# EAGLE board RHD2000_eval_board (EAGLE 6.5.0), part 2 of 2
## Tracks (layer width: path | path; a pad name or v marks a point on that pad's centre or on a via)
+3V3  (via drill 0.25)
  Top 0.381: BRD1.JP2-2 33.93,34.95 34.54,34.95 BRD1.JP2-4 34.75,34.95 35.36,34.95 BRD1.JP2-6 35.56,34.75 35.56,30.07 34.75,29.26 24.18,29.26 24.18,30.48 +3.3V_FPGA_1.1 | BRD1.JP3-9 37.19,81.08 37.8,81.08 BRD1.JP3-11 38,81.08 38.61,81.08 BRD1.JP3-13 38.81,81.08 v38.81,79.65
  Bottom 0.381: v38.81,79.65 44.3,74.17 44.3,65.63 | 44.3,65.63 52.63,65.63 53.65,64.62 77.42,64.62 +3.3V_FPGA_2.1 | 44.3,65.63 31.09,65.63 31.09,37.39 24.18,30.48 +3.3V_FPGA_1.1
+3V3ADC  (via drill 0.25)
  Top 0.381: C20.1 134.31,84.94 v134.31,83.92 134.31,82.7 U10.1 134.11,82.5 134.11,81.89 133.71,81.48 128.83,81.48 128.73,81.58 | C19.1 129.24,84.94 129.24,82.7 U9.1 129.03,82.5 129.03,81.89 128.73,81.58 | C18.1 124.16,84.94 124.16,82.7 U8.1 123.95,82.5 123.95,81.89 123.65,81.58 | C16.1 114,84.94 114,82.7 U6.1 114,82.5 116.43,82.5 116.43,81.89 116.84,81.48 118.87,81.48 | C17.1 119.08,84.94 119.08,82.7 U7.1 118.87,82.5 118.87,81.48 | 123.65,81.58 123.55,81.48 118.87,81.48 | 128.73,81.58 128.63,81.48 123.75,81.48 123.65,81.58 | C15.1 108.92,84.94 v108.92,83.92 108.92,82.7 U5.1 108.71,82.5 108.71,81.89 108.31,81.48 103.63,81.48 | C13.1 98.75,84.94 98.75,82.7 U3.1 98.75,82.5 101.19,82.5 101.19,81.89 101.6,81.48 103.63,81.48 | C14.1 103.83,84.94 103.83,82.7 U4.1 103.63,82.5 103.63,81.48 | 87.58,81.08 84.94,81.08 U2.5 | 87.58,81.08 87.58,79.65 C12.1 | 87.58,81.08 90.83,81.08 90.83,88.8 94.69,92.66 S2.2
  pour Route3: 73.66,97.79 138.43,97.79 138.43,77.47 73.66,77.47
+3V3DAC  (via drill 0.25)
  Top 0.381: 89,30.89 89,31.29 U14.2 | 89,30.89 C32.1 | 89,30.89 U14.1 88.8,30.68 87.99,29.87 87.99,26.21 88.09,26.11 | 89,23.37 89,23.77 U12.2 88.8,23.77 87.99,23.77 87.99,26.01 88.09,26.11 | 89,23.37 89,23.16 U12.1 | 89,23.37 92.66,23.37 C30.1 92.86,23.16 95.5,23.16 95.5,22.55 95.91,22.15 97.54,22.15 97.54,20.52 97.33,20.32 95.5,20.32 95.5,19.3 | 89,27.23 89,27.43 U13.2 | 89,27.23 89,27.03 U13.1 88.8,26.82 88.09,26.11 | 89,27.23 92.66,27.23 C31.1 | U11.1 89,19.51 89,19.91 U11.2 | U11.1 89.2,19.51 92.66,19.51 C29.1 92.86,19.3 95.5,19.3 | 104.55,22.86 104.44,22.96 104.44,29.26 105.26,30.07 C45.1 105.46,30.07 105.46,33.12 112.37,33.12 112.57,32.92 112.57,32.51 112.98,32.11 U22.4 | 104.55,22.86 R13.1 | 95.5,19.3 95.5,18.9 95.91,18.49 104.44,18.49 104.44,22.76 104.55,22.86 | U19.5 111.56,41.66 v113.59,41.66 115.42,41.66 C23.1 115.62,41.45 119.89,37.19 119.89,30.68 120.5,30.07 C46.1 | 89,46.13 89,46.53 U18.2 | 89,46.13 v90.83,46.13 C36.1 | 89,46.13 U18.1 | 89,42.47 89,42.67 U17.2 | 89,42.47 89,42.27 U17.1 | 89,42.47 v90.83,42.47 92.66,42.47 C35.1 | 89,38.61 89,39.01 U16.2 | 89,38.61 89,38.41 U16.1 | 89,38.61 v90.83,38.61 92.66,38.61 C34.1 | U15.2 89,35.15 89,34.75 U15.1 89.2,34.75 v91.03,34.75 92.66,34.75 C33.1 | v111.15,20.32 R14.1 | v117.25,21.54 R15.1 | v122.33,21.54 R16.1 | v126.39,20.32 R17.1 | v132.49,21.54 R18.1 | R19.1 136.55,20.32 v136.55,20.52 | v142.65,21.54 R20.1 | v132.08,33.33 U23.4 | U11.1 88.8,19.3 88.19,18.69 88.19,18.49 76.2,6.5 75.59,6.5 S6.2
  pour Route3: 69.85,1.27 69.85,49.53 153.67,49.53 153.67,1.27
+3V5  (via drill 0.25)
  Top 0.381: U1.6 27.64,89 v29.67,89 30.48,89 C5.1 30.48,90.63 31.5,91.64 31.5,93.67 30.48,94.69 C6.1 | R2.2 20.73,90.42 | 20.73,90.42 C2.1 | v34.54,94.69 35.15,94.08 PORT_A.B6 | v45.31,95.1 45.31,94.08 PORT_B.B6 | v54.66,94.08 55.47,94.08 PORT_C.B6 | v65.02,94.69 65.63,94.08 PORT_D.B6 | v39.42,94.89 40.64,94.89 C7.1 | v50.8,95.91 C8.1 | v59.74,94.89 60.96,94.89 C9.1 | 20.73,90.42 10.97,90.42 10.97,92.66 S10.2
  pour Route3: 8.89,97.79 8.89,83.82 72.39,83.82 72.39,97.79
+5V  (via drill 0.25)
  Top 0.381: U20.2 124.36,44.7 124.36,48.16 C25.1 124.16,48.36 123.04,49.48 | 109.53,46.94 109.53,44.7 U19.3 | 109.53,46.94 111.35,45.11 111.35,44.7 U19.1 | 109.53,46.94 C22.1 109.53,47.14 109.53,49.58 122.94,49.58 123.04,49.48 | 83.21,83.01 83.31,82.91 84.73,82.91 84.73,83.72 U2.1 84.94,83.92 84.94,85.34 85.95,86.36 C11.1 | 83.21,83.01 83.11,83.11 83.11,83.52 82.91,83.72 U2.3 | C3.1 25.81,93.88 25.81,91.64 U1.3 25.81,91.44 25.81,90.42 | 25.81,90.42 27.03,90.42 27.43,90.83 27.43,91.44 U1.1 | BRD1.JP3-5 35.36,81.08 34.75,81.08 BRD1.JP3-3 34.54,81.08 33.93,81.08 BRD1.JP3-1 33.73,81.08 v33.12,81.08 | C1.1 18.9,26.42 13.21,26.42 13.21,26.62 J2.1 | 25.81,90.42 24.38,89 v24.38,81.28 | 83.21,83.01 81.69,81.48 v81.69,76 | v123.14,50.8 123.14,49.58 123.04,49.48
  pour Route3: 1.27,1.27 1.27,81.28 72.39,81.28 72.39,76.2 138.43,76.2 138.43,50.8 68.58,50.8 68.58,1.27
-3V3DAC  (via drill 0.25)
  Top 0.381: v125.58,28.25 124.56,28.25 C47.2 | v131.06,28.04 132.08,27.03 U23.11 | v112.98,27.84 112.98,26.62 U22.11 | 134.31,43.08 137.16,43.08 C28.1 137.16,30.89 C48.2 145.29,22.76 145.29,16.46 148.54,13.21 S1.- | 134.31,43.08 134.31,39.42 R11.2 | 134.31,43.08 U21.5
  Bottom 0.381: v112.98,27.84 113.18,28.04 125.58,28.04 v125.58,28.25 125.78,28.04 v131.06,28.04 132.08,27.03 138.38,27.03 146.3,19.1 146.3,13.21 148.54,13.21 S1.-
-5V_UNREG
  Top 0.381: 132.49,45.92 133.3,45.92 U21.2 | 132.49,45.92 132.49,48.16 C27.1 132.28,48.36 129.44,48.36 L1.2 | 132.49,45.92 U21.3
ADC_!CS!
  Top 0.203: 103.63,80.87 100.79,80.87 100.18,80.26 100.18,80.06 98.75,80.06 U3.6 98.55,80.06 98.55,80.47 97.94,81.08 91.44,81.08 ADC_!CS!.1 91.44,79.86 89,77.42 89,64.62 69.49,45.11 69.49,38.2 50.8,38.2 48.56,35.97 48.56,35.15 48.36,34.95 BRD1.JP2-38 | 103.63,80.87 103.63,80.06 U4.6 | 108.71,80.47 108.71,80.06 U5.6 108.71,80.47 | 108.71,80.47 108.31,80.87 103.63,80.87 | 118.87,80.87 116.84,80.87 116.43,80.47 116.43,80.06 114,80.06 U6.6 113.79,80.06 113.79,81.28 109.53,81.28 108.71,80.47 | 118.87,80.87 118.87,80.06 U7.6 | 123.55,80.87 123.95,80.47 123.95,80.06 U8.6 | 118.87,80.87 123.55,80.87 | 128.63,80.87 129.03,80.47 129.03,80.06 U9.6 | 123.55,80.87 128.63,80.87 | 128.63,80.87 133.71,80.87 134.11,80.47 134.11,80.06 U10.6
ADC_SCLK  (via drill 0.25)
  Top 0.203: U7.4 117.04,79.86 117.04,79.05 112.57,79.05 112.37,79.25 112.37,79.65 112.17,79.86 U6.4 111.96,80.06 v111.15,80.06 | U3.4 96.72,80.06 94.08,80.06 ADC_SCLK.1 93.88,79.86 91.64,77.62 91.64,64.62 76.61,49.58 76.61,44.7 69.7,37.8 51.21,37.8 49.17,35.76 49.17,34.95 BRD1.JP2-40 | v100.99,80.06 101.8,80.06 U4.4 | v106.07,80.06 106.88,80.06 U5.4 | v121.31,80.06 122.12,80.06 U8.4 | v126.39,80.06 127.2,80.06 U9.4 | v131.47,80.06 132.28,80.06 U10.4
  Bottom 0.203: ADC_SCLK.1 94.08,80.06 v100.99,80.06 v106.07,80.06 v111.15,80.06 v121.31,80.06 v126.39,80.06 v131.47,80.06
DAC1_OUT
  Top 0.203: R21.1 107.09,14.43 | 107.09,14.43 107.09,14.22 102.01,14.22 101.6,14.63 101.6,17.68 99.97,17.68 97.54,15.24 R37.1 | 107.09,14.43 R29.2 112.17,9.35 112.17,4.06 118.26,4.06 119.89,5.69 119.89,20.93 116.23,24.59 116.23,27.43 116.64,27.84 116.64,31.7 U22.1
DAC2_OUT
  Top 0.203: 107.9,18.9 106.27,18.9 102.62,15.24 R38.1 | 107.9,18.9 107.9,15.85 108.1,15.65 112.17,15.65 | R22.1 112.17,15.65 | R30.2 112.17,14.43 112.17,15.65 | 107.9,18.9 107.9,20.93 108.1,21.13 108.1,30.89 109.12,31.9 U22.7
GND  (via drill 0.25)
  Top 0.381: 115.42,46.94 112.17,46.94 | 112.17,46.94 111.56,46.94 C22.2 | 115.42,46.94 115.42,44.91 C23.2 | 119.48,48.16 115.42,48.16 115.42,46.94 | 119.48,48.16 122.12,48.16 C25.2 | 110.54,44.7 U19.2 110.34,44.5 110.34,43.89 110.03,43.59 | 110.03,43.59 109.93,43.48 106.68,43.48 C21.2 106.68,44.09 101.8,44.09 | 101.8,44.09 100.38,44.09 C43.2 100.18,44.09 100.18,44.91 95.71,44.91 92.86,47.75 C36.2 | 101.8,44.09 101.8,46.33 100.38,47.75 C44.2 | 112.17,46.94 112.17,43.89 111.76,43.48 110.13,43.48 110.03,43.59 | 134.31,45.92 134.31,48.16 C27.2 | 137.16,45.92 138.58,44.5 138.58,31.09 139.6,30.07 C48.1 139.8,30.07 146.3,23.57 146.3,18.9 148.54,16.66 S1.GND | 137.16,45.92 134.31,45.92 | 134.31,45.92 U21.1 134.11,45.72 134.11,45.11 133.1,44.09 131.47,44.09 131.47,35.76 | 137.16,45.92 C28.2 | C46.2 120.7,28.45 123.34,28.45 123.34,29.06 124.36,30.07 C47.1 124.56,30.07 127,32.51 127,35.97 128.63,37.59 | 124.46,42.77 124.56,42.88 126.8,42.88 126.8,41.86 128.22,40.44 C26.2 128.42,40.23 128.63,40.03 128.63,37.59 | 124.46,42.77 123.55,41.86 U20.4 | 131.47,35.76 128.63,35.76 128.63,37.59 | 131.47,35.76 133.1,35.76 134.11,36.78 R12.1 | 119.48,48.16 119.48,43.48 119.89,43.08 124.36,43.08 124.36,42.88 124.46,42.77 | 100.18,29.67 95.71,29.67 v94.28,31.09 92.86,32.51 C32.2 | 100.18,29.67 100.18,28.85 C39.2 | 100.18,32.92 100.18,32.72 C40.2 100.18,32.92 | 100.18,32.92 100.18,33.53 95.71,33.53 92.86,36.37 C33.2 | 101.3,35.46 101.4,35.36 101.4,34.14 100.18,32.92 | 101.3,35.46 C41.2 | C42.2 106.88,40.23 106.88,38 104.44,35.56 102.41,35.56 | 102.41,35.56 101.4,35.56 101.3,35.46 | 100.18,29.67 102.01,29.67 102.41,30.07 102.41,35.56
  Top 0.381: 96.42,4.17 96.32,4.06 91.44,4.06 91.44,5.08 J1.1 | 96.42,4.17 97.33,5.08 R39.1 97.54,5.08 99.36,6.91 99.36,11.58 102.01,11.58 102.41,11.18 102.41,5.08 R40.1 | 35.15,93.07 PORT_A.T6 35.15,92.86 34.54,92.25 v34.54,87.38 34.54,84.94 33.33,83.72 30.48,83.72 C5.2 | 83.92,85.55 83.92,86.36 C11.2 84.12,86.36 84.12,87.58 | 83.92,85.55 83.92,83.92 U2.2 | 83.92,85.55 82.09,85.55 80.06,83.52 C10.2 | 84.12,87.58 86.77,87.58 87.17,87.17 87.17,83.52 87.58,83.11 C12.2 | 38.61,39.83 38.61,41.05 BRD1.JP2-13 | 38.61,39.83 v38.61,38 38.61,34.95 BRD1.JP2-14 | 38.61,39.83 34.34,39.83 33.93,40.23 33.93,41.05 BRD1.JP2-1 | C31.2 v94.08,27.43 95.5,26.01 100.18,26.01 100.18,24.99 C38.2 | 55.88,36.17 55.68,35.97 55.68,34.95 BRD1.JP2-56 | 55.88,36.17 64.21,36.17 64.21,34.95 BRD1.JP2-78 64.41,34.95 65.02,34.95 BRD1.JP2-80 | 65.63,93.07 PORT_D.T6 65.63,92.86 64.21,92.86 | 64.21,92.86 63.2,92.86 63.2,89.2 62.79,88.8 60.96,88.8 C9.2 | 26.62,91.64 U1.2 26.62,91.85 26.82,92.05 26.82,93.07 27.13,93.37 | 27.13,93.37 27.64,93.88 C3.2 27.64,94.08 26.42,95.3 20.73,95.3 R1.1 20.73,93.88 14.63,93.88 14.63,92.86 S10.1 | C6.2 30.48,93.27 27.23,93.27 27.13,93.37 | 36.58,73.76 38.61,73.76 38.61,74.78 BRD1.JP3-14 | 36.58,73.76 34.34,73.76 33.93,74.17 33.93,74.78 BRD1.JP3-2 | 133.3,82.7 U10.2 133.3,82.91 133.1,83.11 v133.1,83.72 133.1,84.33 132.49,84.94 C20.2 | 128.22,82.7 U9.2 128.22,82.91 128.02,83.11 v128.02,83.72 128.02,84.33 127.41,84.94 C19.2 | 123.14,82.7 U8.2 123.14,82.91 122.94,83.11 v122.94,83.72 122.94,84.33 122.33,84.94 C18.2 | 118.06,82.7 U7.2 118.06,82.91 117.86,83.11 v117.86,83.72 117.86,84.33 117.25,84.94 C17.2
  Top 0.381: 112.98,82.7 U6.2 112.98,82.91 112.78,83.11 v112.78,83.72 112.78,84.33 112.17,84.94 C16.2 | 107.9,82.7 U5.2 107.9,82.91 107.7,83.11 v107.7,83.72 107.7,84.33 107.09,84.94 C15.2 | 102.82,82.7 U4.2 102.82,82.91 102.62,83.11 v102.62,83.72 102.62,84.33 102.01,84.94 C14.2 | 97.74,82.7 U3.2 97.74,82.91 97.54,83.11 v97.54,83.72 97.54,84.33 96.93,84.94 C13.2 | BRD1.JP3-80 65.02,74.98 64.41,74.98 BRD1.JP3-78 64.41,75.18 v64.41,76.2 | 45.31,93.07 PORT_B.T6 45.31,92.86 v45.31,91.85 | 86.36,45.92 U18.8 86.16,45.92 v85.55,45.31 | 86.36,38.41 U16.8 86.36,38.2 86.77,37.8 v86.77,37.59 | 86.36,23.16 U12.8 86.36,22.96 v86.36,22.35 | 86.36,19.3 U11.8 86.16,19.3 v85.14,19.3 | v86.36,26.21 86.36,26.82 U13.8 | v87.38,30.68 86.36,30.68 U14.8 | v86.36,33.73 86.36,34.54 U15.8 | v86.36,41.45 86.36,42.06 U17.8 | v54.66,93.07 55.47,93.07 PORT_C.T6 | v27.64,86.16 27.64,85.14 C4.2 | v91.64,21.13 92.66,21.13 C29.2 | v91.64,24.99 C30.2 | v101.4,21.34 100.38,21.34 C37.2 | v91.64,40.23 C34.2 | v40.64,92.05 C7.2 | v106.48,28.45 105.46,28.45 C45.2 | v91.64,44.09 92.66,44.09 C35.2 | v51,91.24 51,92.86 50.8,93.07 C8.2 | BRD1.JP2-36 47.35,34.75 47.35,30.68 47.14,30.48 GND_1.1 | v47.55,82.7 47.55,81.28 BRD1.JP3-35 | v55.68,82.5 55.68,81.28 BRD1.JP3-55 | C1.2 18.9,29.46 7.32,29.46 7.32,26.82 J2.2 | v36.58,73.56 36.58,73.76 | 64.21,92.86 64.21,95.1 65.63,96.52 78.23,96.52 78.23,92.86 S8.2 | v55.88,36.37 55.88,36.17 | 84.12,87.58 81.89,89.81 81.89,92.66 S8.1 | v96.52,4.06 96.42,4.17
  pour Route2: 1.27,97.79 153.67,97.79 153.67,1.27 1.27,1.27
N$1  (via drill 0.25)
  Top 0.203: v33.73,88.39 33.73,95.91 35.97,95.91 36.58,95.3 36.58,94.08 PORT_A.B4 | v39.22,88.19 39.42,87.99 39.42,81.28 BRD1.JP3-15
  Bottom 0.203: v33.73,88.39 33.93,88.19 v39.22,88.19
N$2  (via drill 0.25)
  Top 0.203: v36.58,91.85 36.58,92.86 PORT_A.T4 | v39.22,90.02 40.23,89 40.23,81.28 BRD1.JP3-17
  Bottom 0.203: v36.58,91.85 38.41,90.02 v39.22,90.02
N$3  (via drill 0.25)
  Top 0.203: v35.76,95.1 35.76,94.08 PORT_A.B5 | v39.22,91.64 41.05,89.81 41.05,81.28 BRD1.JP3-19
  Bottom 0.203: v39.22,91.64 v35.76,95.1
N$4  (via drill 0.25)
  Top 0.203: v35.76,87.17 35.76,92.66 35.97,92.86 PORT_A.T5 | v41.86,87.38 41.86,81.28 BRD1.JP3-21
  Bottom 0.203: v35.76,87.17 35.97,87.38 v41.86,87.38
N$5
  Top 0.203: PORT_A.B1 38.41,93.88 42.67,93.88 42.67,81.28 BRD1.JP3-23
N$6  (via drill 0.25)
  Top 0.203: v38.41,83.31 38.41,92.86 PORT_A.T1 | v43.48,82.5 43.48,81.28 BRD1.JP3-25
  Bottom 0.203: v38.41,83.31 39.22,82.5 v43.48,82.5
N$7
  Top 0.203: PORT_A.B2 37.8,94.08 37.8,94.49 39.01,95.71 43.08,95.71 43.08,83.92 44.3,82.7 44.3,81.28 BRD1.JP3-27
N$8  (via drill 0.25)
  Top 0.203: v37.59,84.73 37.8,84.94 37.8,92.86 PORT_A.T2 | v43.89,84.12 44.91,83.11 44.91,81.28 BRD1.JP3-29
  Bottom 0.203: v37.59,84.73 38.2,84.12 v43.89,84.12
N$9
  Top 0.203: PORT_A.B3 37.19,94.08 37.19,94.89 39.22,96.93 44.5,96.93 44.5,84.53 45.11,83.92 45.11,83.52 45.72,82.91 45.72,81.28 BRD1.JP3-31
N$10  (via drill 0.25)
  Top 0.203: v37.59,82.7 36.78,83.52 36.78,84.94 37.39,85.55 37.39,92.05 37.19,92.25 37.19,92.86 PORT_A.T3 | v40.64,79.65 46.53,79.65 46.53,81.08 BRD1.JP3-33
  Bottom 0.203: v40.64,79.65 v37.59,82.7
N$11  (via drill 0.25)
  Top 0.203: v46.94,95.3 46.74,95.1 46.74,94.08 PORT_B.B4 | v48.77,91.24 48.36,90.83 48.36,81.28 BRD1.JP3-37
  Bottom 0.203: v46.94,95.3 46.94,91.24 v48.77,91.24
N$12  (via drill 0.25)
  Top 0.203: v46.74,84.73 46.74,92.86 PORT_B.T4 | v49.17,84.33 49.17,81.28 BRD1.JP3-39
  Bottom 0.203: v46.74,84.73 47.14,84.33 v49.17,84.33
N$13  (via drill 0.25)
  Top 0.203: v46.13,95.91 46.13,94.08 PORT_B.B5 | v49.99,82.7 49.99,81.28 BRD1.JP3-41
  Route2 0.203: v46.13,95.91 46.13,86.36 49.78,82.7 v49.99,82.7
N$14  (via drill 0.25)
  Top 0.203: v45.92,83.92 45.92,84.73 46.13,84.94 46.13,92.86 PORT_B.T5 | v50.8,83.52 50.8,81.28 BRD1.JP3-43
  Bottom 0.203: v45.92,83.92 46.33,83.52 v50.8,83.52
N$15  (via drill 0.25)
  Top 0.203: v49.38,93.67 49.38,93.88 48.56,93.88 PORT_B.B1 | v52.02,94.49 52.22,94.28 52.22,88.39 51.41,87.58 51.41,83.92 51.61,83.72 51.61,81.28 BRD1.JP3-45
  Bottom 0.203: v49.38,93.67 50.19,94.49 v52.02,94.49
N$16  (via drill 0.25)
  Top 0.203: v50.19,88.39 50.19,92.25 49.78,92.66 49.78,92.86 48.56,92.86 PORT_B.T1 | v52.22,87.38 52.22,81.28 BRD1.JP3-47
  Bottom 0.203: v50.19,88.39 51.21,87.38 v52.22,87.38
N$17  (via drill 0.25)
  Top 0.203: v50.6,84.73 50.6,87.38 51.82,88.59 51.82,93.67 51.61,93.88 50.19,93.88 49.78,94.28 49.78,94.89 48.36,94.89 47.95,94.49 47.95,94.08 PORT_B.B2 | v53.03,82.5 53.03,81.28 BRD1.JP3-49
  Route3 0.203: v50.6,84.73 52.83,82.5 v53.03,82.5
N$18  (via drill 0.25)
  Top 0.203: v49.38,92.05 48.16,92.05 47.95,92.25 47.95,92.86 PORT_B.T2 | v53.65,92.05 53.85,91.85 53.85,81.28 BRD1.JP3-51
  Bottom 0.203: v53.65,92.05 v49.38,92.05
N$19  (via drill 0.25)
  Top 0.203: v53.03,84.53 53.03,87.58 52.83,87.78 52.83,96.72 48.97,96.72 47.75,95.5 47.75,95.1 47.35,94.69 47.35,94.08 PORT_B.B3 | v54.66,82.91 54.66,81.28 BRD1.JP3-53
  Bottom 0.203: v54.66,82.91 v53.03,84.53
N$20  (via drill 0.25)
  Top 0.203: v46.53,82.7 47.55,83.72 47.55,84.73 47.35,84.94 47.35,92.86 PORT_B.T3 | v49.58,79.65 56.29,79.65 56.29,81.08 BRD1.JP3-57
  Bottom 0.203: v49.58,79.65 v46.53,82.7
N$21  (via drill 0.25)
  Top 0.203: v59.54,93.88 58.73,93.88 PORT_C.B1 | v55.47,91.85 54.46,90.83 54.46,84.53 55.68,83.31 57.1,83.31 57.1,81.28 BRD1.JP3-59
  Bottom 0.203: v59.54,93.88 60.35,93.07 60.35,91.85 v55.47,91.85
N$22
  Top 0.203: PORT_C.T1 58.73,92.86 58.73,83.52 57.91,82.7 57.91,81.28 BRD1.JP3-61
N$23  (via drill 0.25)
  Top 0.203: v62.38,89.61 62.38,95.71 59.33,95.71 58.12,94.49 58.12,94.08 PORT_C.B2 | v58.73,82.5 58.73,81.28 BRD1.JP3-63
  Bottom 0.203: v62.38,89.61 62.38,82.5 v58.73,82.5
N$24  (via drill 0.25)
  Top 0.203: v57.91,84.73 58.12,84.94 58.12,92.86 PORT_C.T2 | v59.54,84.12 59.54,81.28 BRD1.JP3-65
  Bottom 0.203: v57.91,84.73 58.52,84.12 v59.54,84.12
N$25  (via drill 0.25)
  Top 0.203: v57.51,95.1 57.51,94.08 PORT_C.B3 | v59.54,92.86 60.35,92.05 60.35,81.28 BRD1.JP3-67
  Bottom 0.203: v57.51,95.1 57.51,92.86 v59.54,92.86
N$26  (via drill 0.25)
  Top 0.203: v56.9,84.73 57.51,85.34 57.51,92.86 PORT_C.T3 | v61.16,83.31 61.16,81.28 BRD1.JP3-69
  Bottom 0.203: v56.9,84.73 58.32,83.31 v61.16,83.31
N$27
  Top 0.203: PORT_D.B1 68.89,93.88 69.9,93.88 69.9,82.5 67.87,80.47 67.87,79.65 67.26,79.05 61.98,79.05 61.98,81.08 BRD1.JP3-71
N$28  (via drill 0.25)
  Top 0.203: v69.09,91.85 69.09,92.66 68.89,92.86 PORT_D.T1 | v63.6,88.39 62.79,87.58 62.79,81.28 BRD1.JP3-73
  Bottom 0.203: v69.09,91.85 67.67,90.42 65.02,90.42 63.6,89 v63.6,88.39
N$29  (via drill 0.25)
  Top 0.203: v68.68,84.73 68.28,85.14 68.28,92.86 PORT_D.T2 | v63.6,82.5 63.6,81.28 BRD1.JP3-75
  Bottom 0.203: v68.68,84.73 66.45,82.5 v63.6,82.5
N$30  (via drill 0.25)
  Top 0.203: v67.87,95.1 67.67,94.89 67.67,94.08 PORT_D.B3 | v64.82,92.05 64.41,91.64 64.41,81.28 BRD1.JP3-77
  Bottom 0.203: v64.82,92.05 v67.87,95.1
N$31  (via drill 0.25)
  Top 0.203: v67.67,84.73 67.67,92.86 PORT_D.T3 | v66.04,83.31 65.23,82.5 65.23,81.28 BRD1.JP3-79
  Bottom 0.203: v67.67,84.73 66.24,83.31 v66.04,83.31
N$32
  Top 0.203: PORT_D.B2 68.28,94.08 68.28,94.49 68.68,94.89 70.31,94.89 70.31,82.3 68.28,80.26 68.28,76.61 65.43,73.76 63.6,73.76 63.6,74.78 BRD1.JP3-76
N$33  (via drill 0.25)
  Top 0.203: v32.11,86.77 32.11,97.74 53.65,97.74 56.69,94.69 56.69,94.08 PORT_C.B4 | v35.56,79.65 39.42,75.79 39.42,74.98 BRD1.JP3-16
  Route2 0.203: v32.11,86.77 32.11,83.11 v35.56,79.65
N$34  (via drill 0.25)
  Top 0.203: v55.27,84.73 56.69,86.16 56.69,92.66 56.9,92.86 PORT_C.T4 | v41.86,73.56 40.44,73.56 40.44,74.78 BRD1.JP3-18
  Route2 0.203: v55.27,84.73 53.85,83.31 51.61,83.31 v41.86,73.56
N$35  (via drill 0.25)
  Top 0.203: v32.92,84.53 32.92,97.33 53.44,97.33 56.08,94.69 56.08,94.08 PORT_C.B5 | v37.8,79.65 41.05,76.4 41.05,74.98 BRD1.JP3-20
  Bottom 0.203: v37.8,79.65 v32.92,84.53
N$36  (via drill 0.25)
  Top 0.203: v55.27,87.38 56.29,88.39 56.29,92.86 PORT_C.T5 | v51.41,78.84 42.06,78.84 42.06,74.98 BRD1.JP3-22
  Bottom 0.203: v55.27,87.38 53.24,85.34 52.83,85.34 51.61,84.12 51.61,78.84 v51.41,78.84
N$37  (via drill 0.25)
  Top 0.203: v66.85,95.1 66.85,94.08 PORT_D.B4 | v28.25,86.97 28.45,86.77 28.45,78.84 34.54,72.75 42.67,72.75 42.67,74.78 BRD1.JP3-24
  Bottom 0.203: v66.85,95.1 60.96,89.2 31.09,89.2 28.85,86.97 v28.25,86.97
N$38  (via drill 0.25)
  Top 0.203: v66.85,81.69 66.85,92.66 67.06,92.86 PORT_D.T4 | v59.33,77.83 46.53,77.83 45.31,76.61 43.69,76.61 43.69,74.98 BRD1.JP3-26
  Bottom 0.203: v66.85,81.69 62.99,77.83 v59.33,77.83
N$39  (via drill 0.25)
  Top 0.203: v68.89,72.75 74.98,78.84 74.98,95.91 66.65,95.91 66.04,95.3 66.04,94.89 66.24,94.69 66.24,94.08 PORT_D.B5 | v45.11,72.75 44.5,73.36 44.5,74.78 BRD1.JP3-28
  Bottom 0.203: v45.11,72.75 v68.89,72.75
N$40  (via drill 0.25)
  Top 0.203: v65.23,89.61 66.24,90.63 66.24,92.66 66.45,92.86 PORT_D.T5 | v49.78,76.2 45.11,76.2 45.11,74.98 BRD1.JP3-30
  Bottom 0.203: v65.23,89.61 65.23,83.31 63.4,83.31 62.79,82.7 62.79,79.65 53.24,79.65 v49.78,76.2
N$41  (via drill 0.25)
  Top 0.203: 86.77,21.74 87.17,22.15 87.17,24.79 | 86.77,21.74 86.36,21.34 U11.5 | 87.17,24.79 86.97,24.99 86.36,24.99 U12.5 | 87.17,24.79 87.17,28.85 86.36,28.85 U13.5 86.16,29.06 85.55,29.06 84.94,29.67 84.94,31.9 85.75,32.72 86.16,32.72 U14.5 86.36,32.92 87.38,32.92 87.38,36.17 86.97,36.58 86.36,36.58 U15.5 86.16,36.58 84.94,36.58 84.94,39.62 85.95,40.64 | 85.95,40.64 85.34,41.25 85.34,43.69 85.75,44.09 | 85.95,40.64 86.16,40.44 U16.5 | 85.75,44.09 86.16,44.09 U17.5 | 85.75,44.09 84.73,45.11 84.73,47.95 86.16,47.95 U18.5 | v40.44,28.85 40.44,31.09 39.62,31.9 39.62,34.75 BRD1.JP2-16 | 86.77,21.74 87.58,20.93 87.58,18.69 86.97,18.09 80.06,18.09 80.06,27.84 DAC_!SYNC!.1
  Bottom 0.203: v40.44,28.85 40.84,28.45 79.45,28.45 79.86,28.04 DAC_!SYNC!.1
N$42  (via drill 0.25)
  Top 0.203: U12.6 86.16,24.59 84.94,24.59 84.33,23.98 84.33,20.73 86.16,20.73 U11.6 86.36,20.52 87.17,20.52 87.17,18.9 86.77,18.49 82.7,18.49 82.7,27.84 DAC_SCLK.1 82.5,28.04 82.5,35.76 84.33,35.76 | 88.19,41.45 88.19,41.66 87.78,42.06 87.78,43.08 87.38,43.48 86.36,43.48 U17.6 | 88.19,41.45 88.19,41.25 87.99,41.05 87.99,39.83 86.36,39.83 U16.6 | v85.14,28.45 85.14,28.25 86.16,28.25 U13.6 | U14.6 86.36,32.11 v87.38,32.11 87.78,32.51 87.78,37.59 93.27,37.59 93.67,38 93.67,39.42 97.13,39.42 97.54,39.83 97.54,41.45 88.19,41.45 | 84.33,35.76 86.16,35.76 U15.6 | 84.33,35.76 84.33,48.56 86.97,48.56 87.17,48.36 87.17,47.55 86.97,47.35 86.36,47.35 U18.6 | v43.08,27.64 40.84,29.87 40.84,31.29 40.23,31.9 40.23,34.75 BRD1.JP2-18
  Bottom 0.203: v87.38,32.11 86.56,31.29 86.56,28.45 v85.14,28.45 84.73,28.04 82.7,28.04 DAC_SCLK.1 82.5,27.84 81.48,26.82 43.89,26.82 v43.08,27.64
N$43  (via drill 0.25)
  Top 0.203: v83.31,33.33 83.31,29.87 83.72,29.46 83.72,20.12 86.16,20.12 U11.7 | v41.05,32.72 41.05,34.75 BRD1.JP2-20
  Bottom 0.203: v83.31,33.33 83.11,33.12 46.53,33.12 45.31,34.34 42.47,34.34 41.05,32.92 v41.05,32.72
N$44  (via drill 0.25)
  Top 0.203: R21.2 108.92,16.66 108.92,20.32 R13.2 108.71,20.32 108.51,20.52 108.51,28.25 v109.73,28.25 | v115.01,30.48 115.01,31.5 115.42,31.9 U22.2
  Bottom 0.203: v115.01,30.48 113.18,28.65 110.13,28.65 v109.73,28.25
N$45  (via drill 0.25)
  Top 0.203: v85.14,23.77 86.16,23.77 U12.7 | v41.66,31.9 41.86,32.11 41.86,34.75 BRD1.JP2-22
  Bottom 0.203: v85.14,23.77 82.5,26.42 41.86,26.42 39.62,28.65 39.62,29.26 39.83,29.26 40.84,30.28 40.84,31.9 v41.66,31.9
N$46  (via drill 0.25)
  Top 0.203: v84.12,30.07 84.12,27.64 86.16,27.64 U13.7 | v42.67,33.53 42.67,34.75 BRD1.JP2-24
  Bottom 0.203: v84.12,30.07 83.72,29.67 47.75,29.67 47.35,29.26 46.53,29.26 45.52,30.28 45.52,31.5 45.11,31.5 43.08,33.53 v42.67,33.53
N$47  (via drill 0.25)
  Top 0.203: v85.75,29.87 85.34,30.28 85.34,31.29 86.16,31.29 U14.7 | v43.48,31.5 43.48,34.75 BRD1.JP2-26
  Bottom 0.203: v85.75,29.87 85.14,29.26 47.95,29.26 47.55,28.85 44.5,28.85 43.28,30.07 43.28,31.5 v43.48,31.5
N$48  (via drill 0.25)
  Top 0.203: v85.34,33.93 85.34,35.15 86.16,35.15 U15.7 | v45.11,33.53 44.5,34.14 44.5,34.75 BRD1.JP2-28
  Bottom 0.203: v85.34,33.93 83.92,32.51 46.53,32.51 45.52,33.53 v45.11,33.53
N$49  (via drill 0.25)
  Top 0.203: v85.75,37.59 85.34,38 85.34,39.01 86.16,39.01 U16.7 | v45.92,36.37 45.11,35.56 45.11,34.95 BRD1.JP2-30
  Bottom 0.203: v85.75,37.59 84.33,39.01 55.27,39.01 52.63,36.37 v45.92,36.37
N$50  (via drill 0.25)
  Top 0.203: v87.38,41.45 87.38,42.88 86.36,42.88 U17.7 | v46.13,31.9 45.92,32.11 45.92,34.75 BRD1.JP2-32
  Bottom 0.203: v87.38,41.45 89.61,39.22 89.61,32.92 85.55,32.92 84.53,31.9 v46.13,31.9
N$51  (via drill 0.25)
  Top 0.203: v87.38,46.74 86.36,46.74 U18.7 | v45.52,39.83 46.74,38.61 46.74,34.95 BRD1.JP2-34
  Bottom 0.203: v87.38,46.74 86.77,46.13 51.82,46.13 v45.52,39.83
N$52  (via drill 0.25)
  Top 0.203: v133.1,78.84 133.1,79.65 133.3,79.86 U10.5 | v47.55,73.56 47.55,46.13 45.11,43.69 45.11,41.25 BRD1.JP2-29
  Bottom 0.203: v133.1,78.84 131.67,77.42 73.56,77.42 73.15,77.01 51.61,77.01 48.16,73.56 v47.55,73.56
N$53
  Top 0.203: R30.1 112.17,12.6 114.4,10.36 114.4,6.5 DAC_OUT.2
N$54  (via drill 0.25)
  Top 0.203: v77.42,45.31 96.32,64.21 96.32,64.82 98.96,67.46 98.96,75.18 102.62,78.84 102.62,79.65 102.82,79.86 U4.5 | v52.02,45.31 50.8,44.09 50.8,41.25 BRD1.JP2-43
  Bottom 0.203: v52.02,45.31 v77.42,45.31
N$55  (via drill 0.25)
  Top 0.203: v106.07,57.51 128.02,79.45 128.02,79.65 128.22,79.86 U9.5 | v45.92,42.47 45.92,41.25 BRD1.JP2-31
  Bottom 0.203: v106.07,57.51 104.44,55.88 82.7,55.88 81.69,54.86 58.32,54.86 v45.92,42.47
N$56  (via drill 0.25)
  Top 0.203: v100.99,57.51 122.94,79.45 122.94,79.65 123.14,79.86 U8.5 | v47.55,45.11 46.74,44.3 46.74,41.25 BRD1.JP2-33
  Bottom 0.203: v100.99,57.51 99.77,56.29 82.5,56.29 81.48,55.27 57.71,55.27 v47.55,45.11
N$57  (via drill 0.25)
  Top 0.203: v97.13,57.51 117.86,78.23 117.86,79.65 118.06,79.86 U7.5 | v49.17,55.68 48.36,54.86 48.36,41.25 BRD1.JP2-37
  Bottom 0.203: v97.13,57.51 96.32,56.69 82.3,56.69 81.28,55.68 v49.17,55.68
N$58  (via drill 0.25)
  Top 0.203: v76,41.45 98.96,64.41 98.96,65.02 109.73,75.79 109.73,80.87 112.57,80.87 112.78,80.67 112.78,80.26 112.98,80.06 U6.5 | v53.85,39.01 49.17,39.01 49.17,41.05 BRD1.JP2-39
  Bottom 0.203: v76,41.45 75.59,41.05 56.69,41.05 54.66,39.01 v53.85,39.01
N$59  (via drill 0.25)
  Top 0.203: v101.8,72.34 107.7,78.23 107.7,79.65 107.9,79.86 U5.5 | v61.98,67.87 49.99,55.88 49.99,41.25 BRD1.JP2-41
  Bottom 0.203: v101.8,72.34 98.55,69.09 64.21,69.09 62.99,67.87 v61.98,67.87
N$60  (via drill 0.25)
  Top 0.203: v77.62,48.16 93.88,64.41 93.88,75.18 97.54,78.84 97.54,79.65 97.74,79.86 U3.5 | v54.66,46.94 51.61,43.89 51.61,41.25 BRD1.JP2-45
  Bottom 0.203: v77.62,48.16 76.4,46.94 v54.66,46.94
N$61
  Top 0.203: R31.1 117.25,12.6 117.86,11.99 117.86,6.5 DAC_OUT.3
N$62
  Top 0.203: R32.1 122.33,12.6 121.51,11.79 121.51,6.5 DAC_OUT.4
N$63
  Top 0.203: R33.1 127.41,12.6 124.97,10.16 124.97,6.5 DAC_OUT.5
N$64
  Top 0.203: R34.1 132.49,12.6 128.42,8.53 128.42,6.5 DAC_OUT.6
N$65
  Top 0.203: R35.1 137.57,12.6 132.08,7.11 132.08,6.5 DAC_OUT.7
N$66
  Top 0.203: R36.1 142.65,12.6 136.55,6.5 135.53,6.5 DAC_OUT.8
N$67
  Top 0.203: U11.3 89,20.73 89,21.13 U11.4 89,21.34 89,21.95 93.47,21.95 93.67,21.74 93.67,21.34 96.52,21.34 R3.2
N$68  (via drill 0.25)
  Top 0.203: v68.68,56.9 68.68,44.7 65.23,41.25 BRD1.JP2-79 | v121.11,60.35 148.54,87.78 148.54,88.39 3.3V_DIGITAL_IN.16
  Bottom 0.203: v68.68,56.9 70.51,58.73 119.48,58.73 v121.11,60.35
N$69  (via drill 0.25)
  Top 0.203: v64.41,56.49 64.41,41.25 BRD1.JP2-77 | v132.08,66.85 146.3,81.08 146.3,82.7 148.54,84.94 3.3V_DIGITAL_IN.15
  Bottom 0.203: v64.41,56.49 64.82,56.08 81.08,56.08 83.31,58.32 123.55,58.32 v132.08,66.85
N$70  (via drill 0.25)
  Top 0.203: v63.6,49.78 63.6,41.25 BRD1.JP2-75
  Bottom 0.203: v63.6,49.78 65.63,51.82 144.07,51.82 147.12,48.77 150.16,48.77 151.59,50.19 151.59,81.28 148.74,81.28 3.3V_DIGITAL_IN.14
N$71  (via drill 0.25)
  Top 0.203: v62.59,68.68 62.79,68.48 62.79,41.25 BRD1.JP2-73
  Bottom 0.203: v62.59,68.68 62.59,70.71 92.66,70.71 96.72,74.78 96.72,77.01 147.73,77.01 148.54,77.83 3.3V_DIGITAL_IN.13
N$72  (via drill 0.25)
  Top 0.203: v76.2,60.35 69.09,53.24 69.09,44.5 65.63,41.05 65.63,40.03 62.38,40.03 61.98,40.44 61.98,41.05 BRD1.JP2-71
  Bottom 0.203: v76.2,60.35 76.61,60.76 95.3,60.76 99.16,64.62 99.16,65.84 100.79,65.84 101.8,64.82 101.8,63.6 111.56,63.6 122.33,74.37 148.54,74.37 3.3V_DIGITAL_IN.12
N$73  (via drill 0.25)
  Top 0.203: v61.77,52.22 61.16,51.61 61.16,41.25 BRD1.JP2-69
  Bottom 0.203: v61.77,52.22 63.2,53.65 146.1,53.65 148.13,55.68 149.96,55.68 151.18,56.9 151.18,70.92 148.74,70.92 3.3V_DIGITAL_IN.11
N$74  (via drill 0.25)
  Top 0.203: v60.55,52.22 60.55,41.45 60.35,41.25 BRD1.JP2-67
  Bottom 0.203: v60.55,52.22 62.38,54.05 143.05,54.05 148.13,59.13 149.96,59.13 150.77,59.94 150.77,67.46 148.74,67.46 3.3V_DIGITAL_IN.10
N$75  (via drill 0.25)
  Top 0.203: v59.54,56.49 59.54,41.25 BRD1.JP2-65
  Bottom 0.203: v59.54,56.49 62.18,59.13 107.7,59.13 116.23,67.67 144.88,67.67 148.54,64.01 3.3V_DIGITAL_IN.9
N$76  (via drill 0.25)
  Top 0.203: v58.73,52.22 58.73,41.25 BRD1.JP2-63
  Bottom 0.203: v58.73,52.22 58.73,54.46 83.72,54.46 84.73,55.47 143.66,55.47 148.54,60.35 3.3V_DIGITAL_IN.8
N$77  (via drill 0.25)
  Top 0.203: v68.07,39.83 68.07,39.01 59.33,39.01 58.12,40.23 58.12,40.84 57.91,41.05 BRD1.JP2-61 | v76.61,40.64 83.92,47.95 83.92,48.77 86.77,51.61 124.16,51.61 124.16,50.8 124.77,50.19 136.14,50.19 142.85,56.9 148.54,56.9 3.3V_DIGITAL_IN.7
  Bottom 0.203: v68.07,39.83 68.89,40.64 v76.61,40.64
N$78  (via drill 0.25)
  Top 0.203: v57.3,51 57.3,41.25 BRD1.JP2-59
  Bottom 0.203: v57.3,51 57.71,51.41 61.98,51.41 63.8,53.24 148.34,53.24 148.54,53.44 3.3V_DIGITAL_IN.6
N$79  (via drill 0.25)
  Top 0.203: v56.49,49.58 56.49,41.25 BRD1.JP2-57
  Bottom 0.203: v56.49,49.58 57.1,50.19 61.37,50.19 63.4,52.22 146.3,52.22 148.54,49.99 3.3V_DIGITAL_IN.5
N$80  (via drill 0.25)
  Top 0.203: v54.46,39.83 54.46,40.84 54.66,41.05 BRD1.JP2-53 | v135.13,46.94 138.79,50.6 138.79,51.21 139.4,51.82 146.3,51.82 146.3,48.77 148.54,46.53 3.3V_DIGITAL_IN.4
  Bottom 0.203: v54.46,39.83 56.9,42.27 90.02,42.27 90.63,41.66 96.52,41.66 101.8,46.94 v135.13,46.94
N$81  (via drill 0.25)
  Top 0.203: v55.68,47.75 55.68,46.94 54.05,45.31 54.05,41.25 BRD1.JP2-51
  Bottom 0.203: v55.68,47.75 56.9,48.97 94.89,48.97 95.5,49.58 135.13,49.58 136.96,51.41 141.22,51.41 146.3,46.33 146.3,43.08 148.54,43.08 3.3V_DIGITAL_IN.3
N$82  (via drill 0.25)
  Top 0.203: v53.24,39.83 53.24,41.05 BRD1.JP2-49 | v136.96,47.75 139.19,49.99 139.19,51 139.6,51.41 145.9,51.41 145.9,42.27 148.54,39.62 3.3V_DIGITAL_IN.2
  Bottom 0.203: v53.24,39.83 56.69,43.28 97.54,43.28 102.01,47.75 v136.96,47.75
N$83  (via drill 0.25)
  Top 0.203: v52.43,42.47 52.43,41.25 BRD1.JP2-47 | v135.53,48.97 138.79,52.22 150.77,52.22 150.77,38.2 148.74,36.17 3.3V_DIGITAL_IN.1
  Bottom 0.203: v52.43,42.47 54.46,44.5 91.03,44.5 95.5,48.97 v135.53,48.97
N$84
  Top 0.203: R56.2 63.6,22.35 63.6,34.75 BRD1.JP2-76
N$85
  Top 0.203: R55.2 66.04,16.26 62.79,19.51 62.79,34.75 BRD1.JP2-74
N$86
  Top 0.203: R54.2 62.18,16.26 61.98,16.46 61.98,34.75 BRD1.JP2-72
N$87
  Top 0.203: R53.2 58.52,16.26 60.96,18.69 60.96,34.75 BRD1.JP2-70
N$88
  Top 0.203: R52.2 54.66,16.26 60.15,21.74 60.15,34.75 BRD1.JP2-68
N$89
  Top 0.203: R51.2 50.8,16.26 56.49,21.95 59.33,21.95 59.33,34.75 BRD1.JP2-66
N$90
  Top 0.203: R50.2 53.24,22.35 57.91,22.35 57.91,33.53 58.52,34.14 58.52,34.75 BRD1.JP2-64
N$91
  Top 0.203: R49.2 43.28,16.26 49.78,22.76 57.51,22.76 57.51,33.93 57.71,34.14 57.71,34.75 BRD1.JP2-62
N$92
  Top 0.203: R48.2 39.42,16.26 46.33,23.16 57.1,23.16 57.1,34.75 BRD1.JP2-60
N$93  (via drill 0.25)
  Top 0.203: v37.8,18.69 37.8,18.49 35.56,16.26 R47.2 | v46.53,23.98 56.29,23.98 56.29,34.75 BRD1.JP2-58
  Bottom 0.203: v37.8,18.69 43.08,23.98 v46.53,23.98
N$94  (via drill 0.25)
  Top 0.203: R46.2 42.47,26.82 44.09,26.82 v44.09,27.64 | v54.66,27.64 54.66,34.75 BRD1.JP2-54
  Bottom 0.203: v54.66,27.64 v44.09,27.64
N$95  (via drill 0.25)
  Top 0.203: v30.48,18.69 28.04,16.26 R45.2 | v47.14,24.79 49.58,24.79 52.02,27.23 53.85,27.23 53.85,34.75 BRD1.JP2-52
  Bottom 0.203: v30.48,18.69 36.58,24.79 v47.14,24.79
N$96  (via drill 0.25)
  Top 0.203: v26.62,18.69 24.18,16.26 R44.2 | v47.95,25.6 48.97,25.6 51,27.64 53.03,27.64 53.03,34.75 BRD1.JP2-50
  Bottom 0.203: v26.62,18.69 33.53,25.6 v47.95,25.6
N$97  (via drill 0.25)
  Top 0.203: v21.54,16.26 20.32,16.26 R43.2 | v39.22,17.88 49.38,28.04 52.22,28.04 52.22,34.75 BRD1.JP2-48
  Bottom 0.203: v21.54,16.26 23.16,17.88 v39.22,17.88
N$98
  Top 0.203: R42.2 16.46,16.26 16.05,16.26 15.44,16.87 11.79,16.87 11.79,15.44 11.99,15.24 14.02,15.24 14.02,4.88 14.83,4.06 34.95,4.06 34.95,12.19 38.41,15.65 38.41,18.29 48.56,28.45 51.41,28.45 51.41,34.75 BRD1.JP2-46
N$99
  Top 0.203: R41.2 12.8,16.05 15.65,16.05 15.65,15.44 15.85,15.24 34.54,15.24 34.54,16.66 46.74,28.85 50.6,28.85 50.6,34.75 BRD1.JP2-44
N$100
  Top 0.203: U10.3 132.28,82.7 131.67,83.31 131.67,92.66 ADC_IN.1
N$101
  Top 0.203: U9.3 127.2,82.7 126.59,83.31 126.59,91.24 128.02,92.66 ADC_IN.2
N$102
  Top 0.203: U8.3 122.12,82.7 121.51,83.31 121.51,89.61 124.56,92.66 ADC_IN.3
N$103
  Top 0.203: U7.3 117.04,82.7 116.43,83.31 116.43,87.99 121.11,92.66 ADC_IN.4
N$104
  Top 0.203: U6.3 111.96,82.7 111.35,83.31 111.35,86.36 117.65,92.66 ADC_IN.5
N$105
  Top 0.203: U5.3 106.88,82.7 106.27,83.31 106.27,85.75 110.54,90.02 114,90.02 114,92.66 ADC_IN.6
N$106
  Top 0.203: U4.3 101.8,82.7 101.19,83.31 101.19,85.75 105.87,90.42 110.54,90.42 110.54,92.66 ADC_IN.7
N$107
  Top 0.203: U3.3 96.72,82.7 96.11,83.31 96.11,85.75 103.02,92.66 107.09,92.66 ADC_IN.8
N$108
  Top 0.203: U2.4 82.91,81.08 83.72,80.26 83.72,74.57 82.91,73.76 81.08,73.76 81.08,75.59 80.06,76.61 80.06,81.69 C10.1
N$109
  Top 0.203: R3.1 96.52,19.51 100.18,19.51 C37.1 100.38,19.3 103.63,22.55 103.63,34.14 113.18,34.14 113.79,33.53 113.79,32.51 114.2,32.11 U22.3
N$110
  Top 0.203: R37.2 95.71,15.24 98.15,12.8 98.15,10.16 C49.1
N$111
  Top 0.203: U13.3 89,28.45 89,28.85 U13.4 89,29.06 89,29.67 93.27,29.67 93.67,29.26 93.67,28.85 96.52,28.85 R5.2
N$112
  Top 0.203: U14.3 89,32.11 89,32.72 U14.4 89,32.92 89,33.53 93.27,33.53 93.67,33.12 93.67,32.72 96.52,32.72 R6.2
N$113
  Top 0.203: R29.1 107.09,12.6 110.74,8.94 110.74,6.5 DAC_OUT.1
N$114
  Top 0.203: U12.3 89,24.59 89,24.99 U12.4 89,25.2 89,25.81 93.47,25.81 93.67,25.6 93.67,24.99 R4.2
N$115
  Top 0.203: U15.3 89,35.97 89,36.37 U15.4 89,36.58 89,37.19 93.47,37.19 94.08,36.58 96.52,36.58 R7.2
N$116
  Top 0.203: U16.3 89,39.83 89,40.23 U16.4 89,40.44 89,41.05 93.47,41.05 93.67,40.84 93.67,40.23 R8.2
N$117
  Top 0.203: U17.3 89,43.69 89,44.09 U17.4 89,44.3 89,44.91 93.27,44.91 93.67,44.5 93.67,44.09 96.52,44.09 R9.2
N$118
  Top 0.203: U18.3 89,47.35 89,47.95 U18.4 89,48.16 89,48.77 93.27,48.77 93.67,48.36 93.67,47.95 96.52,47.95 R10.2
N$119  (via drill 0.25)
  Top 0.203: R22.2 114,16.66 114,20.32 R14.2 113.79,20.32 113.79,21.54 v113.18,22.15 | v111.56,23.77 111.56,25.2 111.15,25.6 111.15,27.43 110.95,27.64 110.95,31.5 110.54,31.9 U22.6
  Bottom 0.203: v113.18,22.15 v111.56,23.77
N$120  (via drill 0.25)
  Top 0.203: R4.1 96.52,23.37 100.18,23.37 C38.1 100.38,23.37 102.41,25.4 102.41,28.85 v102.82,29.26 | v111.76,29.67 U22.5
  Bottom 0.203: v111.76,29.67 111.35,29.26 v102.82,29.26
N$121
  Top 0.203: R38.2 100.79,15.24 101.19,14.83 101.19,13.41 104.44,10.16 C50.1
N$122  (via drill 0.25)
  Top 0.203: R5.1 96.52,27.23 100.18,27.23 C39.1 100.38,27.23 100.38,27.43 v101.6,27.43 | v111.76,27.84 U22.10
  Bottom 0.203: v111.76,27.84 111.35,27.43 v101.6,27.43
N$123  (via drill 0.25)
  Top 0.203: R23.2 119.08,16.66 119.08,20.32 R15.2 118.87,20.32 118.87,20.93 v116.03,23.77 | v110.54,25.2 110.54,26.42 U22.9
  Bottom 0.203: v110.54,25.2 111.15,24.59 115.21,24.59 v116.03,23.77
N$124  (via drill 0.25)
  Top 0.203: R6.1 C40.1 100.38,30.89 100.38,30.48 v101.6,30.48 | v113.79,30.28 113.79,27.03 114.2,26.62 U22.12
  Bottom 0.203: v113.79,30.28 113.59,30.48 v101.6,30.48
N$125
  Top 0.203: R31.2 117.25,14.43 R23.1 117.25,16.66 116.23,17.68 116.23,22.96 111.35,22.96 109.73,24.59 109.73,26.01 109.32,26.42 U22.8
N$126  (via drill 0.25)
  Top 0.203: R7.1 96.52,34.75 v99.16,34.75 100.18,34.75 C41.1 | v133.1,33.33 133.1,32.31 133.3,32.11 U23.3
  Bottom 0.203: v133.1,33.33 131.67,34.75 v99.16,34.75
N$127
  Top 0.203: C50.2 101.19,10.16 101.19,5.49 100.79,5.08 R40.2 100.58,5.08 100.58,3.25 87.99,3.25 84.12,7.11 J1.3
N$128  (via drill 0.25)
  Top 0.203: R8.1 96.52,38.61 100.18,38.61 C42.1 100.38,38.41 v106.07,38.41 | v127.81,35.56 130.25,33.12 130.25,32.51 130.66,32.11 U23.5
  Bottom 0.203: v127.81,35.56 124.97,38.41 v106.07,38.41
N$129
  Top 0.203: R32.2 122.33,14.43 R24.1 122.33,16.66 121.51,17.48 121.51,21.74 116.84,26.42 U22.14
N$130  (via drill 0.25)
  Top 0.203: R9.1 96.52,42.47 100.18,42.47 C43.1 100.38,42.27 100.38,41.45 106.88,41.45 v114.4,33.93 | v130.25,29.67 130.25,27.03 130.66,26.62 U23.10
  Bottom 0.203: v130.25,29.67 125.98,33.93 v114.4,33.93
N$131  (via drill 0.25)
  Top 0.203: R25.2 129.24,16.66 129.24,20.32 R17.2 129.03,20.32 129.03,20.73 127.61,22.15 127.61,28.85 v129.44,28.85 | v134.31,29.67 134.31,31.7 134.52,31.9 U23.2
  Bottom 0.203: v134.31,29.67 133.5,28.85 v129.44,28.85
N$132  (via drill 0.25)
  Top 0.203: R10.1 C44.1 100.38,46.13 100.38,45.72 v100.99,45.11 | v133.5,30.28 133.5,26.62 U23.12
  Bottom 0.203: v133.5,30.28 133.5,32.72 133.91,33.12 133.91,45.11 v100.99,45.11
N$133  (via drill 0.25)
  Top 0.203: R33.2 127.41,14.43 R25.1 v127.41,19.1 | v137.36,26.21 136.55,27.03 136.55,31.29 135.94,31.9 U23.1
  Bottom 0.203: v137.36,26.21 137.36,19.1 v127.41,19.1
N$134
  Top 0.203: R26.2 134.31,16.66 134.31,20.32 R18.2 134.11,20.32 134.11,20.93 132.69,22.35 132.69,28.25 130.05,30.89 130.05,31.5 129.64,31.9 U23.6
N$135
  Top 0.203: R34.2 132.49,14.43 132.49,15.65 | R26.1 132.49,15.65 | 132.49,15.65 128.42,15.65 128.22,15.85 128.22,20.93 127.2,21.95 127.2,30.89 128.22,31.9 U23.7
N$136  (via drill 0.25)
  Top 0.203: R27.2 139.4,16.66 139.4,20.32 R19.2 139.19,20.32 v135.53,23.98 | v130.05,25.2 130.05,26.01 129.64,26.42 U23.9
  Bottom 0.203: v130.05,25.2 131.27,23.98 v135.53,23.98
N$137
  Top 0.203: R35.2 137.57,14.43 137.57,15.65 | R27.1 137.57,15.65 | 137.57,15.65 133.5,15.65 133.3,15.85 133.3,17.88 128.83,22.35 128.83,26.01 128.42,26.42 U23.8
N$138
  Top 0.203: R20.2 144.47,20.32 144.47,16.66 R28.2 144.47,16.46 145.29,15.65 145.29,11.79 143.87,11.79 143.46,12.19 143.46,13.61 140.61,13.61 138.38,15.85 138.38,17.68 134.72,21.34 134.72,26.42 U23.13
N$139
  Top 0.203: R36.2 143.87,13.21 143.87,15.24 142.65,16.46 R28.1 142.65,16.66 141.83,17.48 141.83,20.52 135.94,26.42 U23.14
N$140
  Top 0.203: R39.2 95.5,5.08 94.89,5.69 94.89,10.16 C49.2 94.69,10.16 94.69,11.38 91.44,14.63 J1.2
N$141
  Top 0.203: C21.1 106.68,41.86 109.53,41.86 U19.4
N$142
  Top 0.203: R24.2 124.16,16.66 124.16,20.32 R16.2 123.95,20.32 123.95,20.93 119.28,25.6 119.28,33.12 116.43,33.12 116.23,32.92 116.23,30.89 115.82,30.48 115.82,26.82 115.62,26.62 U22.13
N$143
  Top 0.203: C4.1 25.81,88.8 U1.4
N$144
  Top 0.203: 22.55,91.44 22.55,93.88 R1.2 | U1.5 26.62,88.8 26.62,82.5 24.59,80.47 22.55,80.47 22.55,87.58 C2.2 22.55,87.78 22.55,91.44 | 22.55,91.44 R2.1
N$145
  Top 0.381: U20.5 125.37,41.66 124.36,40.64 120.7,40.64 120.7,42.06 C24.1
N$146
  Top 0.381: U20.3 123.34,44.5 120.7,44.5 120.7,44.3 C24.2
N$147
  Top 0.203: R41.1 12.6,14.22 11.99,13.61 11.99,6.5 3.3V_DIGITAL_OUT.1
N$148
  Top 0.203: R42.1 16.46,14.22 15.44,13.21 15.44,6.5 3.3V_DIGITAL_OUT.2
N$149
  Top 0.203: R43.1 20.32,14.22 18.9,12.8 18.9,6.5 3.3V_DIGITAL_OUT.3
N$150
  Top 0.203: U21.4 132.49,43.08 R11.1 R12.2
N$151
  Top 0.203: R44.1 22.35,12.6 22.35,6.5 3.3V_DIGITAL_OUT.4
N$152
  Top 0.203: R45.1 27.84,14.22 26.01,12.39 26.01,6.5 3.3V_DIGITAL_OUT.5
N$153
  Top 0.203: R46.1 31.7,14.22 29.46,11.99 29.46,6.5 3.3V_DIGITAL_OUT.6
N$154
  Top 0.203: R47.1 35.56,14.22 32.92,11.58 32.92,6.5 3.3V_DIGITAL_OUT.7
N$155
  Top 0.203: R48.1 36.37,11.38 36.37,6.5 3.3V_DIGITAL_OUT.8
N$156
  Top 0.203: R49.1 43.08,14.22 40.03,11.18 40.03,6.5 3.3V_DIGITAL_OUT.9
N$157
  Top 0.203: R50.1 46.94,14.22 43.48,10.77 43.48,6.5 3.3V_DIGITAL_OUT.10
N$158
  Top 0.203: R51.1 50.8,14.22 46.94,10.36 46.94,6.5 3.3V_DIGITAL_OUT.11
N$159
  Top 0.203: R52.1 50.39,10.16 50.39,6.5 3.3V_DIGITAL_OUT.12
N$160
  Top 0.203: R53.1 58.32,14.22 54.05,9.96 54.05,6.5 3.3V_DIGITAL_OUT.13
N$161
  Top 0.203: R54.1 62.18,14.22 57.51,9.55 57.51,6.5 3.3V_DIGITAL_OUT.14
N$162
  Top 0.203: R55.1 66.04,14.22 60.96,9.14 60.96,6.5 3.3V_DIGITAL_OUT.15
N$163
  Top 0.203: R56.1 64.41,8.94 64.41,6.5 3.3V_DIGITAL_OUT.16
N$164
  Top 0.381: 127.2,44.5 128.22,44.5 128.22,43.69 C26.1 | 127.2,44.5 125.58,44.5 U20.1 | 127.2,44.5 127.2,48.16 L1.1
N$165  (via drill 0.25)
  Top 0.203: v39.42,37.39 39.42,41.05 BRD1.JP2-15
  Bottom 0.203: v39.42,37.39 37.59,35.56 31.9,35.56 26.82,30.48 G16-L9P.1
N$166  (via drill 0.25)
  Top 0.203: v40.23,39.22 40.23,41.05 BRD1.JP2-17
  Bottom 0.203: v40.23,39.22 39.83,38.81 33.33,38.81 25.6,31.09 25.6,29.26 27.84,29.26 29.06,30.48 G16-L9N.1
N$167  (via drill 0.25)
  Top 0.203: v41.05,39.83 41.05,41.05 BRD1.JP2-19
  Bottom 0.203: v41.05,39.83 41.05,35.15 36.58,35.15 31.9,30.48 H19-L34P.1
N$168
  Top 0.203: BRD1.JP2-21 41.86,41.25 41.66,41.45 41.66,42.06 41.45,42.27 33.33,42.27 33.33,31.29 34.14,30.48 H18-L34N.1
N$169  (via drill 0.25)
  Top 0.203: v42.47,39.83 42.47,40.84 42.67,41.05 BRD1.JP2-23
  Bottom 0.203: v42.47,39.83 42.47,35.15 41.66,35.15 36.98,30.48 F16-L10P.1
N$170  (via drill 0.25)
  Top 0.203: v43.28,39.22 43.28,40.84 43.48,41.05 BRD1.JP2-25
  Bottom 0.203: v43.28,39.22 43.28,34.75 42.06,34.75 39.42,32.11 39.42,30.48 F17-L10N.1
N$171  (via drill 0.25)
  Top 0.203: v44.3,36.37 44.3,41.05 BRD1.JP2-27
  Route2 0.203: v44.3,36.37 44.3,33.33 42.06,31.09 42.06,30.48 J17-L36P.1
N$172
  Top 0.203: BRD1.JP2-42 49.78,34.75 49.78,31.7 47.35,29.26 44.5,29.26 44.5,30.48 U20-L51P.1
N$173  (via drill 0.25)
  Top 0.203: v45.92,71.93 45.92,74.78 BRD1.JP3-32 | v63.6,67.06 79.86,67.06 79.86,64.82 D9-L7P.1
  Bottom 0.203: v45.92,71.93 50.8,67.06 v63.6,67.06
N$174  (via drill 0.25)
  Top 0.203: v46.74,64.82 46.74,74.78 BRD1.JP3-34
  Bottom 0.203: v46.74,64.82 52.63,64.82 53.44,64.01 76.61,64.01 77.01,63.6 81.48,63.6 82.5,64.62 C8-L7P.1
N$175  (via drill 0.25)
  Top 0.381: v36.17,82.5 36.17,81.28 BRD1.JP3-7
  Bottom 0.381: v36.17,82.5 33.33,85.34 8.74,85.34 7.72,86.36 +1.8V_FPGA.1
N$176  (via drill 0.25)
  Top 0.203: v48.36,68.48 48.36,74.78 BRD1.JP3-38
  Bottom 0.203: v48.36,68.48 50.6,66.24 83.52,66.24 84.94,64.82 D10-L33P.1
N$177  (via drill 0.25)
  Top 0.203: v49.17,64.01 49.17,74.78 BRD1.JP3-40
  Bottom 0.203: v49.17,64.01 52.83,64.01 53.24,63.6 76.4,63.6 76.81,63.2 86.16,63.2 87.58,64.62 C10-L33N.1
N$178  (via drill 0.25)
  Top 0.203: v49.99,63.2 49.99,74.78 BRD1.JP3-42
  Bottom 0.203: v49.99,63.2 76.2,63.2 76.61,62.79 88.19,62.79 D11-L36P.1
N$179  (via drill 0.25)
  Top 0.203: v51,62.38 51,63.4 50.8,63.6 50.8,74.78 BRD1.JP3-44
  Bottom 0.203: v51,62.38 51.41,62.79 75.18,62.79 75.59,62.38 90.42,62.38 92.66,64.62 C12-L36N.1
N$180  (via drill 0.25)
  Top 0.203: v51.82,61.77 51.82,62.59 51.61,62.79 51.61,74.78 BRD1.JP3-46
  Bottom 0.203: v51.82,61.77 52.43,62.38 74.98,62.38 75.39,61.98 92.46,61.98 D15-L62P.1
N$181  (via drill 0.25)
  Top 0.203: v53.03,61.57 52.43,62.18 52.43,74.78 BRD1.JP3-48
  Bottom 0.203: v53.03,61.57 53.44,61.98 74.78,61.98 75.59,61.16 94.28,61.16 97.74,64.62 C16-L62N.1
N$182  (via drill 0.25)
  Top 0.203: v54.25,61.16 54.25,61.37 53.24,62.38 53.24,74.78 BRD1.JP3-50
  Bottom 0.203: v54.25,61.16 55.88,59.54 95.1,59.54 B6-L4P.1
N$183  (via drill 0.25)
  Top 0.203: v54.05,65.43 54.05,74.78 BRD1.JP3-52
  Bottom 0.203: v54.05,65.43 54.46,65.84 83.11,65.84 83.92,65.02 83.92,63.6 85.55,63.6 86.56,64.62 86.56,66.24 101.4,66.24 A6-L4P.1
N$184  (via drill 0.25)
  Top 0.203: v54.86,76.2 54.86,74.98 BRD1.JP3-54
  Bottom 0.203: v54.86,76.2 56.08,74.98 77.42,74.98 C7-L5P.1
N$185  (via drill 0.25)
  Top 0.381: BRD1.JP3-6 35.36,74.98 34.75,74.98 BRD1.JP3-4 34.54,74.98 34.54,76.2 29.06,81.69 v29.06,88.19
  Bottom 0.381: v29.06,88.19 28.45,88.8 7.72,88.8 +1.2V_FPGA.1
N$186  (via drill 0.25)
  Top 0.203: v56.49,76.2 56.49,74.98 BRD1.JP3-58
  Bottom 0.203: v56.49,76.2 57.3,75.39 76.4,75.39 77.01,76 78.84,76 79.86,74.98 A7-L5N.1
N$187  (via drill 0.25)
  Top 0.203: v57.1,73.56 57.1,74.78 BRD1.JP3-60
  Bottom 0.203: v57.1,73.56 57.91,74.37 76.4,74.37 77.01,73.76 81.48,73.76 82.5,74.78 C9-L8P.1
N$188  (via drill 0.25)
  Top 0.203: v58.12,73.56 58.12,74.57 57.91,74.78 BRD1.JP3-62
  Bottom 0.203: v58.12,73.56 76.61,73.56 76.81,73.36 83.52,73.36 A9-L8N.1
N$189
  Top 0.203: BRD1.JP3-64 58.73,74.78 58.93,74.57 58.93,71.12 60.15,69.9 61.37,69.9 61.98,70.51 62.99,70.51 62.99,69.49 65.02,67.46 81.08,67.46 81.08,68.28 87.58,74.78 B12-L37P.1
N$190  (via drill 0.25)
  Top 0.203: v59.74,71.32 59.74,74.57 59.54,74.78 BRD1.JP3-66
  Bottom 0.203: v59.74,71.32 59.94,71.53 86.77,71.53 A12-L37N.1
N$191  (via drill 0.25)
  Top 0.203: v60.55,70.71 60.55,74.57 60.35,74.78 BRD1.JP3-68
  Bottom 0.203: v60.55,70.71 60.96,71.12 89,71.12 92.66,74.78 B14-L50P.1
N$192  (via drill 0.25)
  Top 0.203: v65.84,76.2 65.84,77.01 62.59,77.01 61.37,75.79 61.37,75.18 61.16,74.98 BRD1.JP3-70
  Bottom 0.203: v65.84,76.2 66.24,76.61 81.28,76.61 81.48,76.81 93.27,76.81 95.1,74.98 A14-L50N.1
N$193  (via drill 0.25)
  Top 0.203: v63.8,69.7 63.8,70.31 61.98,72.14 61.98,74.78 BRD1.JP3-72
  Bottom 0.203: v63.8,69.7 64.21,70.1 93.07,70.1 97.74,74.78 B16-L63P.1
N$194  (via drill 0.25)
  Top 0.203: v68.48,68.28 62.79,73.97 62.79,74.78 BRD1.JP3-74
  Bottom 0.203: v68.48,68.28 68.89,68.68 99.16,68.68 102.62,72.14 102.62,73.76 101.4,73.76 100.38,74.78 A16-L63N.1

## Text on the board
tPlace: A | B | C | D | ADC Inputs (0 - +3.3V) | RHD2000 SPI Interfaces | Intan Technologies | RHD2000 EVALUATION BOARD | Version 1.0 | http://www.intantech.com | Opal Kelly XEM6010 | 3.3V Digital Input Lines | PJ-102AH | 3.3V Digital Output Lines | DAC Outputs (-3.3V - +3.3V) | Audio Line Out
